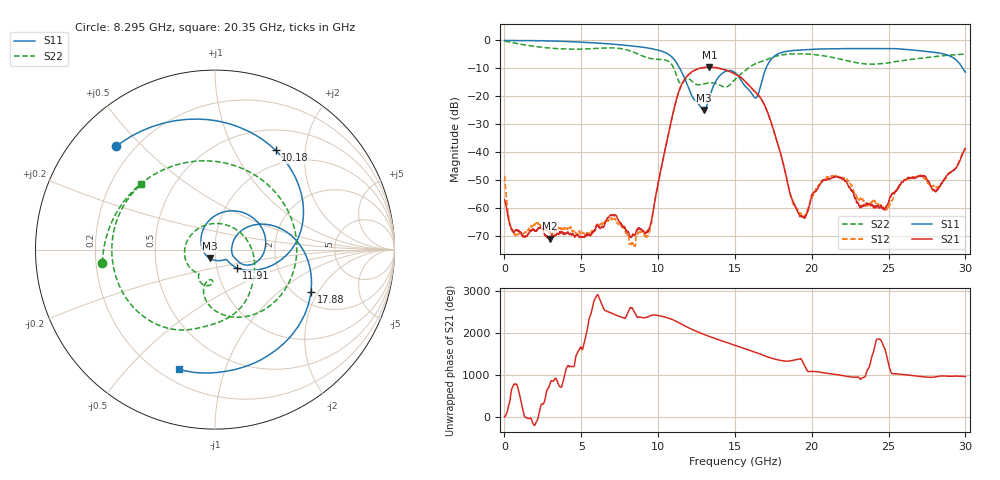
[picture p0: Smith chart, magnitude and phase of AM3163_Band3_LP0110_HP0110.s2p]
!Agilent Technologies,E8364B,MY43040894,A.07.50.67
!Agilent E8364B: A.07.50.67
!Date: Thursday, August 20, 2020 11:05:24
!Correction: S11(Full 2 Port(1,2))
!S21(Full 2 Port(1,2))
!S12(Full 2 Port(1,2))
!S22(Full 2 Port(1,2))
!S2P File: Measurements: S11, S21, S12, S22:
# Hz S  dB  R 50
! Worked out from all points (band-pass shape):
!   3201 points, 10 MHz to 30 GHz, reference 50 ohm
!   highest |S21| = -9.59 dB at 13.34 GHz (marker M1); lowest = -71.1 dB at 2.943 GHz (marker M2)
!   |S21| within 3 dB of the highest: 11.93 GHz to 15.19 GHz (3.268 GHz wide, 24.1 % of centre)
!   lowest |S11| = -24.9 dB at 12.96 GHz (marker M3), VSWR 1.12, Z = 47 - j4.65 ohm
!   |S11| at or under -10 dB: 11.41 GHz to 17.02 GHz (5.614 GHz wide, 39.5 % of centre); 29.82 GHz to end of sweep
!   |S22| runs from -16.8 to -0.3 dB; largest |S21 - S12| = 0.005
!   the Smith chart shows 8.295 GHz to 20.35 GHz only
!   S11 on the Smith chart (normalised r, x): 8.295 GHz: 0.13, +0.42; 10.18 GHz: 0.78, +1.49; 11.91 GHz: 1.24, -0.26; 17.88 GHz: 2.40, -1.74; 20.35 GHz: 0.27, -0.71
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1e7  -0.02 -2.1  -57.17 -2.3  -48.52 143.1  -0.26 -6.3
4.5985e8  -0.05 -12.6  -67.77 -79.0  -67.71 101.4  -0.75 -39.9
1.162741e9  -0.05 -31.7  -69.93 -131.4  -69.65 -1.5  -1.49 -92.4
2.943397e9  -0.20 -79.8  -71.08 39.5  -68.97 6.0  -2.75 161.4
5.014581e9  -0.65 -134.1  -70.37 -167.8  -69.06 -36.1  -3.13 52.5
7.095138e9  -1.37 169.9  -62.71 -65.7  -64.59 -67.9  -2.69 -76.7
8.294738e9  -1.98 133.7  -70.39 84.5  -72.69 -110.9  -3.99 -173.4
9.372503e9  -2.75 95.0  -68.21 -129.3  -69.28 55.3  -6.34 78.7
1.000979e10  -3.50 67.0  -50.88 -102.6  -51.23 -103.2  -6.80 10.6
1.017848e10  -3.77 58.6  -46.34 -112.6  -46.56 -114.8  -6.84 -7.1
1.191228e10  -16.09 -40.2  -12.67 -22.5  -12.75 -22.1  -13.69 -105.0
1.296193e10  -24.91 -119.8  -9.74 169.9  -9.79 170.2  -15.61 -130.9
1.333681e10  -20.55 146.5  -9.59 118.0  -9.66 118.2  -15.24 -146.8
1.5005e10  -11.58 -8.3  -12.02 -93.7  -12.01 -93.4  -13.98 4.3
1.635455e10  -20.65 2.2  -18.55 97.4  -18.76 97.5  -8.32 -77.7
1.788217e10  -4.66 -24.0  -38.80 -86.8  -38.77 -84.9  -5.38 -132.9
1.917548e10  -3.45 -74.4  -62.55 -61.2  -61.58 -62.0  -4.81 -178.9
2.000958e10  -3.19 -98.0  -55.51 5.1  -56.65 4.3  -5.00 151.2
2.034697e10  -3.13 -106.8  -53.41 -5.3  -52.93 -8.0  -5.20 138.6
2.290549e10  -2.94 -165.9  -57.95 -136.8  -55.71 -128.4  -8.00 21.9
2.500479e10  -3.00 145.0  -57.84 163.7  -59.66 -100.1  -8.05 -86.1
3e10  -11.38 -19.4  -38.87 -120.1  -38.60 -115.2  -4.91 104.0
